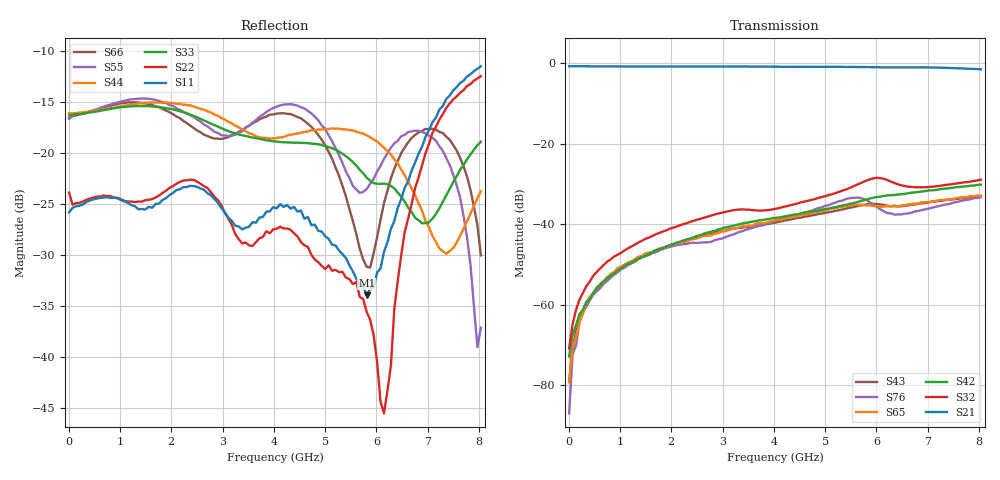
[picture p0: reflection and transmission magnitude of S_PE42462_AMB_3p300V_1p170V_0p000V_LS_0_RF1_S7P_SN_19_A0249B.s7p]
! Device ID: PE42462
! File Path: z:\PE42462\DataSheet S-parameter-6T\AMB\3p300\LS_0_RF1\PE42462_AMB_3p300V_1p170V_0p000V_LS_0_RF1_S7P_SN_19_A0249B.s7p
! Serial: 19
! Lot: A0249B
! Temp: AMB
! VDD: 3.300
! VSS: 0.000
! Control_Hi: 1.170
! Control_Lo: 0.000
! Logic State: LS_0_RF1
! Port 1:
! Port 2:
! Port 3:
! Port 4:
! Port 5:
! Port 6:
! Port 7:
! ThroughPath:1-2
! IDD: 0.0001047097
! ISS/IDD2: -7.1e-009
! IDMM3/IDD3: -2.56e-007
! Comment:
#  Hz  S  RI  R  50
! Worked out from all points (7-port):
!   120 points, 10 MHz to 8.037 GHz, reference 50 ohm
!   strongest paths, dB at 10 MHz, 2.034 GHz, 4.057 GHz, 6.08 GHz, 8.037 GHz:
!     S21: -0.7, -0.8, -0.8, -1.0, -1.5
!     S32: -70.9, -40.9, -36.1, -28.5, -28.9
!     S42: -72.9, -45.0, -38.4, -33.1, -30.2
!     S65: -79.3, -44.9, -39.0, -35.7, -32.9
!     S76: -87.1, -45.5, -39.0, -36.3, -33.3
!     S43: -79.2, -45.0, -39.5, -35.1, -33.0
!   lowest |S11| = -34.0 dB at 5.811 GHz (marker M1), VSWR 1.04, Z = 48.6 - j1.42 ohm
!   |S11| at or under -10 dB: start of sweep to end of sweep
